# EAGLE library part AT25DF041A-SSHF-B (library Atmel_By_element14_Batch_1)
4-megabit Minimum SPI Serial Flash Memory
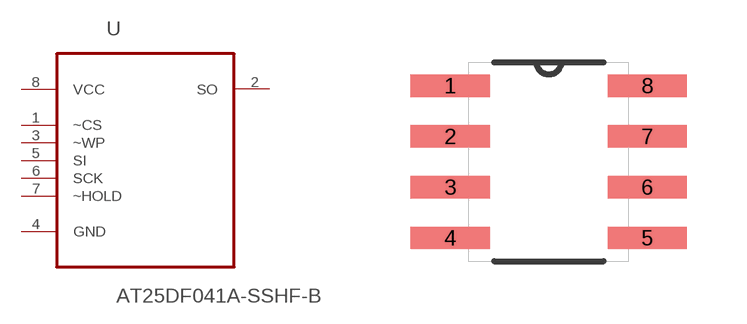
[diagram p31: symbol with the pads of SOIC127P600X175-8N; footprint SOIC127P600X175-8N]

Designator prefix U

## AT25DF041A-SSHF-B (MPN: AT25DF041A-SSHF-B; OC_FARNELL: 1636622; OC_NEWARK: 03P2050; PACKAGE: SOIC-8; SUPPLIER: Atmel)  [SOIC127P600X175-8N]
1  ~CS  in
2  SO  out
3  ~WP  in
4  GND  pas
5  SI  in
6  SCK  in
7  ~HOLD  in
8  VCC  pwr

## Footprint SOIC127P600X175-8N (pad centres in mm)
smd 1.981 x 0.559: 1 -2.464,1.905; 2 -2.464,0.635; 3 -2.464,-0.635; 4 -2.464,-1.905; 5 2.464,-1.905; 6 2.464,-0.635; 7 2.464,0.635; 8 2.464,1.905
